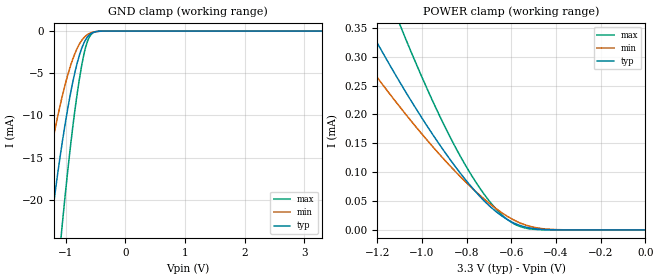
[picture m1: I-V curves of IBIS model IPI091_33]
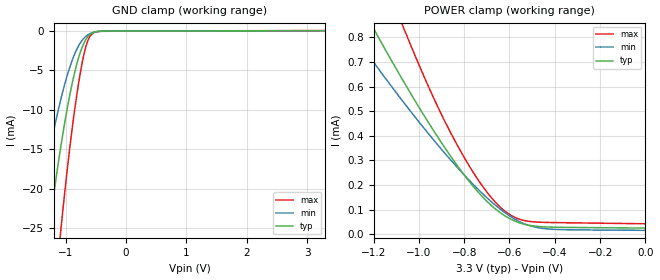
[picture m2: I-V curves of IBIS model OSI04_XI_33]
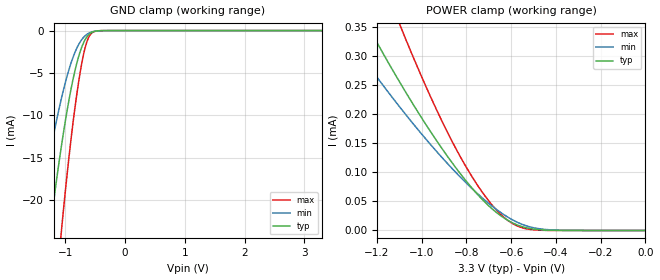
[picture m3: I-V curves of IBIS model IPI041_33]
| TEXAS INSTRUMENTS INCORPORATED
| Connectivity Solutions Group
| IBIS Model of TL16C752C_3.3V
| 752C_3.3V
| This file contains package information for the following:
|  QFP 32-pin (QFP) package as [Component] 752C_3.3V
| This device can be powered at the following Vccs:
|  3.3 Volt Vcc
| This file provides unique models under the [Model Selector] for each Vcc.
| For operation at a specific Vcc, select the appropriate model after each
| [Model Selector] keyword.
[IBIS Ver]   3.2
[Comment char]  |_char
[File Name]   752c_rhb_3_3v.ibs
[File Rev]   1 | a
[Date]   December 5, 2007
[Source]   Data created from TI-SPICE simulations at TI-CONN.
[Notes]   The following is an IBIS list for the 752C_3.3V.
   Please contact s-ly@ti.com with questions and
   comments concerning CONN IBIS models.
[Disclaimer] Property of Texas Instruments Incorporated.  Unauthorized
   reproduction and/or distribution is strictly prohibited.
   This product is protected under copyright law.
   Created  2003, (C) Copyright  2003, Texas Instruments
   Incorporated, All Rights Reserved
   UNLESS THERE IS A SIGNED, WRITTEN AGREEMENT TO THE
   CONTRARY, TEXAS INSTRUMENTS (TI) IS PROVIDING THE IBIS
   MODELS  AND WITHOUT ANY WARRANTY, EXPRESSED OR
   IMPLIED.  TI assumes no liability for:
   1) the accuracy of the IBIS models provided to your
   company;
   2) the proper functioning of these IBIS Models in your
   design or for any resulting applications; or
   3) infringement of patents, copyrights or intellectual
   property rights resulting from your use of these IBIS
   models.
   TI provides IBIS Models as a service to our customers.
   You and your company shall not distribute, sell or give
   these models to anyone else without prior written
   permission from TI.
   TI reserves the right to make changes to our products or
   to discontinue any semiconductor product or service
   without notice, and advises our customers to obtain the
   latest version of relevant information to verify, before
   placing orders, that the information being relied on is
   current.
   Please be aware that your receipt and use of the IBIS
   information provided shall serve as acceptance of these
   terms and conditions.  If you do not accept these terms,
   you should return or destroy the IBIS models and any
   other accompanying information immediately.
| Component 752C_3.3V_QFP 32-pin QFP
[Component]   752C_RHB_3.3V
[Manufacturer]   Texas Instruments, Inc.
[Package]
|   typ   min   max
R_pkg   0.03169   0.03002   0.03704
L_pkg   2.02289n   1.83543n   2.62435n
C_pkg   0.52087p   0.46196p   0.61212p
[Pin]   signal_name   model_name   R_pin   L_pin   C_pin
1   D6   IPI04_OPJ43   0.03132   1.96376n   0.50826p
2   D7   IPI04_OPJ43   0.03166   2.03022n   0.52764p
3   RXB   IPI041   0.03222   2.12197n   0.55702p
4   RXA   IPI041   0.03290   2.21862n   0.57989p
5   TXA   OPJ430   0.03010   1.83593n   0.46505p
6   TXB   OPJ430   0.03096   1.92107n   0.49718p
7   CSA   IPI041   0.03104   1.92183n   0.49798p
8   CSB   IPI041   0.03110   1.96691n   0.51031p
9   XTAL1   OSI04_XI   0.03077   1.83703n   0.47632p
10   XTAL2   OSI04   0.03175   1.92839n   0.50935p
11   IOW   IPI041   0.03007   1.83565n   0.46474p
12   GND   GND   0.03265   2.22076n   0.58208p
13   IOR   IPI041   0.03002   1.83657n   0.46196p
14   RTSB   OPJ430   0.03190   2.11324n   0.55339p
15   CTSB   IPI041   0.03704   2.62435n   0.54475p
16   A2   IPI041   0.03147   1.97163n   0.51867p
17   A1   IPI041   0.03142   1.92513n   0.50753p
18   A0   IPI041   0.03060   1.83543n   0.47574p
19   INTB   OPJ430   0.03159   2.04484n   0.53228p
20   INTA   OPJ430   0.03117   1.96768n   0.51149p
21   RTSA   OPJ430   0.03153   2.03432n   0.53110p
22   DTRA   OPJ430   0.03280   2.22331n   0.58366p
23   DTRB   OPJ430   0.03352   2.34940n   0.60960p
24   RESET   IPI091   0.03188   1.96764n   0.51741p
25   CTSA   IPI041   0.03373   2.35631n   0.61212p
26   VCC   POWER   0.03224   2.13122n   0.55769p
27   D0   IPI04_OPJ43   0.03191   2.05000n   0.53623p
28   D1   IPI04_OPJ43   0.03138   1.96454n   0.50911p
29   D2   IPI04_OPJ43   0.03132   1.92758n   0.49950p
30   D3   IPI04_OPJ43   0.03043   1.84011n   0.46416p
31   D4   IPI04_OPJ43   0.03039   1.83956n   0.46402p
32   D5   IPI04_OPJ43   0.03129   1.92740n   0.49881p
| Model IPI091
[Model Selector]   IPI091
IPI091_33   3.3 volt Vcc
| Model OSI04_XI
[Model Selector]   OSI04_XI
OSI04_XI_33   3.3 volt Vcc
| Model IPI041
[Model Selector]   IPI041
IPI041_33   3.3 volt Vcc
| Model IPI04_OPJ43
[Model Selector]   IPI04_OPJ43
IPI04_OPJ43_33   3.3 volt Vcc
| Model OPJ430
[Model Selector]   OPJ430
OPJ430_33   3.3 volt Vcc
| Model OSI04
[Model Selector]   OSI04
OSI04_33   3.3 volt Vcc
| Models and submodels in the file (6): IPI091_33 (Input), OSI04_XI_33 (Input), IPI041_33 (Input), IPI04_OPJ43_33 (I/O), OPJ430_33 (3-state), OSI04_33 (3-state)
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[Model]   IPI091_33
Model_type  Input
Vinl = 0
Vinh = 3.3
| variable   typ   min   max
C_comp   1.07pF   0.95pF   1.20pF
[Temperature Range]   40   125   -40
| Ambient temperature   25   110   -40
[Voltage range]   3.3   3   3.6
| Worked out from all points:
|   GND clamp passes 1 mA (typ) near -0.66 V on its own axis
|   POWER clamp passes 1 mA (typ) near -2.03 V on its own axis
[GND Clamp]
| IPI091_33
|   Voltage   I(typ)   I(min)   I(max)
-3.3V     -184.1mA   -131.7mA   -253.5mA
-1.485V   -37.43mA   -23.94mA   -59.12mA
-1.28V    -24.78mA   -15.34mA   -40.66mA
-1.25V    -23.07mA   -14.2mA    -38.11mA
-1.075V   -13.97mA   -8.224mA   -24.19mA
-1.06V    -13.26mA   -7.774mA   -23.08mA
-940mV    -8.152mA   -4.58mA    -14.87mA
-805mV    -3.718mA   -2.005mA   -7.28mA
-700mV    -1.488mA   -825uA     -2.909mA
-600mV    -421.4uA   -273uA     -659.6uA
-400mV    -8.531uA   -12.92uA   -6.748uA
3.3V      251.6pA    69.15nA    65.83pA
[POWER Clamp]
| IPI091_33
|   Voltage   I(typ)   I(min)   I(max)
-3.3V     2.289mA    1.713mA    3.253mA
-1.35V    432uA      344.6uA    613.8uA
-1.225V   341.4uA    277.2uA    481uA
-1.11V    263.3uA    218.6uA    366.4uA
-1.075V   240.6uA    201.5uA    333.1uA
-930mV    152.9uA    134.7uA    205.1uA
-805mV    87.01uA    83.43uA    112uA
-700mV    42.42uA    46.59uA    50.87uA
-620mV    18.66uA    24.18uA    18.85uA
-540mV    5.375uA    9.01uA     3.55uA
-445mV    638.3nA    1.643uA    187.2nA
-47.99fV  251.6pA    2.2nA      73.1pA
[Model]   OSI04_XI_33
Model_type  Input
Vinl = 0
Vinh = 3.3
| variable   typ   min   max
C_comp   1.85pF   1.15pF   2.42pF
[Temperature Range]   40   125   -40
| Ambient temperature   25   110   -40
[Voltage range]   3.3   3   3.6
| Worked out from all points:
|   GND clamp passes 1 mA (typ) near -0.66 V on its own axis
|   POWER clamp passes 1 mA (typ) near -1.30 V on its own axis
[GND Clamp]
| OSI04_XI_33
|   Voltage   I(typ)   I(min)   I(max)
-3.3V     -187.4mA   -133.6mA   -258.6mA
-1.52V    -40.73mA   -26.12mA   -63.96mA
-1.48V    -38.05mA   -24.28mA   -60.12mA
-1.275V   -25.2mA    -15.59mA   -41.32mA
-1.095V   -15.43mA   -9.17mA    -26.46mA
-1.07V    -14.21mA   -8.387mA   -24.55mA
-935mV    -8.294mA   -4.704mA   -15.09mA
-800mV    -3.791mA   -2.104mA   -7.36mA
-695mV    -1.529mA   -912.1uA   -2.917mA
-600mV    -479.4uA   -361uA     -744.5uA
-390mV    -35.35uA   -32.95uA   -52.71uA
3.3V      25.17uA    17.8uA     39.06uA
[POWER Clamp]
| OSI04_XI_33
|   Voltage   I(typ)   I(min)   I(max)
-3.3V     5.294mA    3.984mA    7.572mA
-1.3V     1.007mA    827.6uA    1.402mA
-1.195V   827.7uA    692.7uA    1.14mA
-1.075V   632.4uA    545.1uA    855.7uA
-1.04V    577.7uA    503.5uA    776.7uA
-915mV    392.6uA    361.2uA    514.8uA
-815mV    259.4uA    256uA      336.3uA
-720mV    152.9uA    166.1uA    196.6uA
-625mV    77.8uA     91.06uA    97.45uA
-555mV    46.18uA    50.98uA    60.77uA
-455mV    30.55uA    24.01uA    48.59uA
-47.99fV  25.17uA    16.02uA    42.63uA
[Model]   IPI041_33
Model_type  Input
Vinl = 0
Vinh = 3.3
| variable   typ   min   max
C_comp   1.08pF   0.95pF   1.21pF
[Temperature Range]   40   125   -40
| Ambient temperature   25   110   -40
[Voltage range]   3.3   3   3.6
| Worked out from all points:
|   GND clamp passes 1 mA (typ) near -0.66 V on its own axis
|   POWER clamp passes 1 mA (typ) near -2.03 V on its own axis
[GND Clamp]
| IPI041_33
|   Voltage   I(typ)   I(min)   I(max)
-3.3V     -184.1mA   -131.7mA   -253.5mA
-1.485V   -37.43mA   -23.94mA   -59.12mA
-1.28V    -24.78mA   -15.34mA   -40.66mA
-1.25V    -23.07mA   -14.2mA    -38.11mA
-1.075V   -13.97mA   -8.224mA   -24.19mA
-1.06V    -13.26mA   -7.774mA   -23.08mA
-940mV    -8.152mA   -4.58mA    -14.87mA
-805mV    -3.718mA   -2.005mA   -7.28mA
-700mV    -1.488mA   -825uA     -2.909mA
-600mV    -421.4uA   -273uA     -659.6uA
-400mV    -8.531uA   -12.92uA   -6.748uA
3.3V      251.6pA    69.15nA    65.83pA
[POWER Clamp]
| IPI041_33
|   Voltage   I(typ)   I(min)   I(max)
-3.3V     2.289mA    1.713mA    3.253mA
-1.35V    432uA      344.6uA    613.8uA
-1.225V   341.4uA    277.2uA    481uA
-1.11V    263.3uA    218.6uA    366.4uA
-1.075V   240.6uA    201.5uA    333.1uA
-930mV    152.9uA    134.7uA    205.1uA
-805mV    87.01uA    83.43uA    112uA
-700mV    42.42uA    46.59uA    50.87uA
-620mV    18.66uA    24.18uA    18.85uA
-540mV    5.375uA    9.01uA     3.55uA
-445mV    638.3nA    1.643uA    187.2nA
-47.99fV  251.6pA    2.2nA      73.1pA
